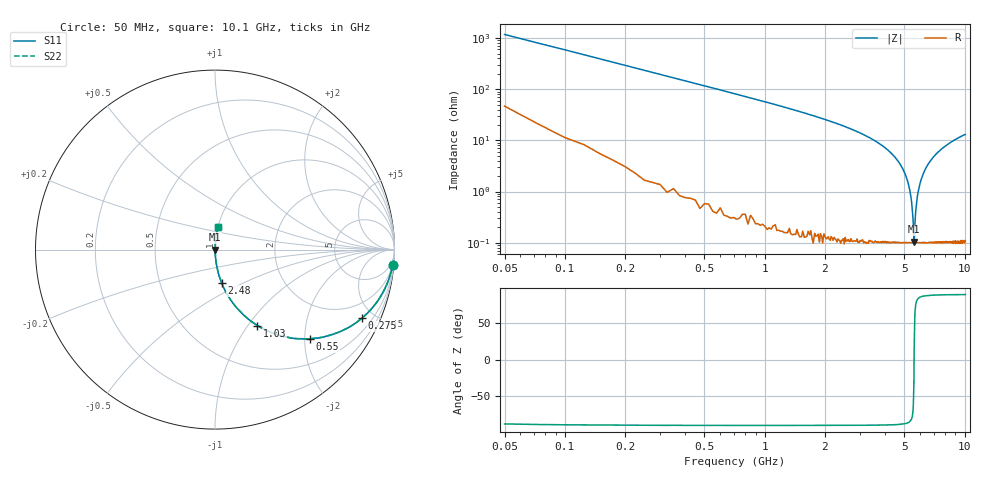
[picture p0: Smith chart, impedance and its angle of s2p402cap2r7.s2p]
! AVX Thin Film Operation		Date: April 2003
! Description: Accu-P® Series, Thin Film, SMD, RF Capacitor
! Part Number: 04025J2R7ABS
! 50 MHz  -  10.05 GHz
! Serial Measurements
# hz S db R 50
!	S11		S21		S12		S22
!	dB	Phase	dB	Phase	dB	Phase	dB	Phase
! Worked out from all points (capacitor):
!   400 points, 50 MHz to 10.1 GHz, reference 50 ohm
!   read as one part in series: C = 2.7 pF near 100 MHz
!   lowest |Z| = 105 mohm at 5.6 GHz (marker M1)
!   series resonance near 5.594 GHz, so ESL is about 300 pH
!   S11 on the Smith chart (normalised r, x): 50 MHz: 2, -24; 275 MHz: 1.03, -4.27; 550 MHz: 1.01, -2.12; 1.03 GHz: 1.00, -1.11; 2.48 GHz: 1.00, -0.38; 10.1 GHz: 1.00, +0.26
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5e7  -0.06 -4.8  -21.50 82.9  -21.50 82.9  -0.06 -4.8
1.25e8  -0.22 -11.9  -13.70 77.1  -13.70 77.1  -0.22 -11.9
2.75e8  -0.88 -25.0  -7.49 64.6  -7.49 64.6  -0.88 -25.0
5.5e8  -2.78 -43.2  -3.30 46.6  -3.30 46.6  -2.78 -43.2
1.03e9  -6.28 -60.8  -1.18 29.0  -1.18 29.0  -6.28 -60.8
1.73e9  -10.60 -72.6  -0.41 17.2  -0.41 17.2  -10.60 -72.6
2.48e9  -14.50 -78.8  -0.17 10.8  -0.17 10.8  -14.50 -78.8
3.4e9  -19.30 -83.2  -0.06 6.2  -0.06 6.2  -19.30 -83.2
4.33e9  -25.20 -85.8  -0.02 3.1  -0.02 3.1  -25.20 -85.8
5.08e9  -33.80 -86.0  -0.01 1.2  -0.01 1.2  -33.80 -86.0
5.28e9  -38.20 -84.7  -0.01 0.7  -0.01 0.7  -38.20 -84.7
5.43e9  -43.80 -80.7  -0.01 0.4  -0.01 0.4  -43.80 -80.7
5.53e9  -51.30 -68.4  -0.01 0.1  -0.01 0.1  -51.30 -68.4
5.58e9  -58.50 -32.9  -0.01 0.0  -0.01 0.0  -58.50 -32.9
5.6e9  -59.60 16.5  -0.01 -0.0  -0.01 -0.0  -59.60 16.5
5.65e9  -52.40 65.1  -0.01 -0.1  -0.01 -0.1  -52.40 65.1
5.7e9  -47.60 75.8  -0.01 -0.2  -0.01 -0.2  -47.60 75.8
5.9e9  -38.90 84.3  -0.01 -0.6  -0.01 -0.6  -38.90 84.3
6.2e9  -33.20 86.1  -0.01 -1.2  -0.01 -1.2  -33.20 86.1
6.75e9  -28.00 86.3  -0.02 -2.3  -0.02 -2.3  -28.00 86.3
8.43e9  -21.10 84.3  -0.04 -5.1  -0.04 -5.1  -21.10 84.3
1.01e10  -17.80 82.1  -0.08 -7.4  -0.08 -7.4  -17.80 82.1
